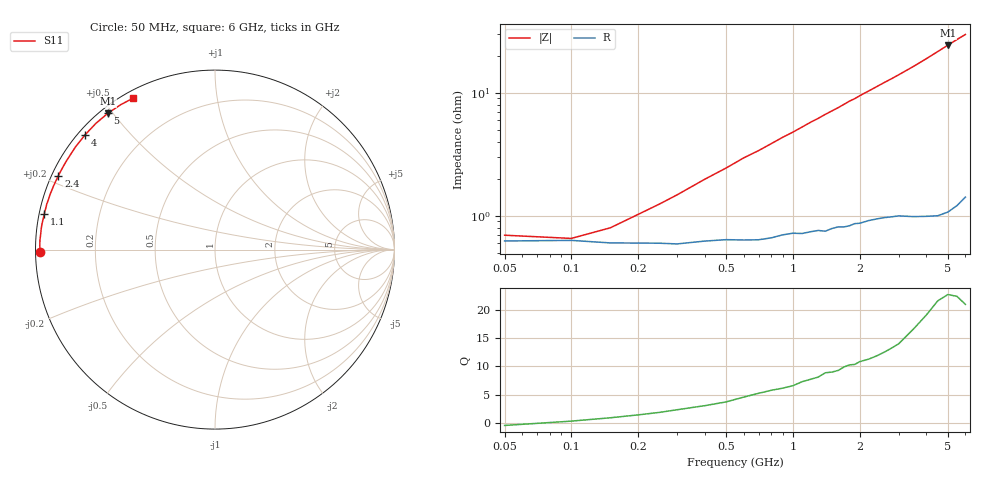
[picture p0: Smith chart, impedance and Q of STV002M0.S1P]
! SIEMENS Discrete & RF Semiconductors
! BA892
! Si PIN Diode in SCD-80
! IF = 2 mA
! S-Parameters:  September  1997
# GHz  S  MA  R  50
!  f  S11
! GHz  MAG  ANG
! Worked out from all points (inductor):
!   34 points, 50 MHz to 6 GHz, reference 50 ohm
!   read as one part to ground: L = 753 pH near 400 MHz
!   highest Q = 22.4 at 5 GHz (marker M1), where L = 774 pH
!   S11 on the Smith chart (normalised r, x): 50 MHz: 0.01, -0.01; 1.1 GHz: 0.01, +0.10; 2.4 GHz: 0.02, +0.22; 4 GHz: 0.02, +0.38; 5 GHz: 0.02, +0.49; 6 GHz: 0.03, +0.59
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0.05  0.9754 -179.3
0.1  0.9752 179.6
0.15  0.9763 178.8
0.2  0.9764 178.1
0.3  0.9768 176.9
0.6  0.9751 173.4
0.7  0.975 172.4
0.8  0.9741 171.3
0.9  0.9727 170.2
1  0.9719 169.2
1.1  0.9721 168.1
1.2  0.9712 167.0
1.3  0.9706 166.0
1.4  0.971 164.9
1.6  0.9688 162.9
1.8  0.9683 160.7
1.9  0.9672 159.8
2  0.9671 158.7
2.4  0.9648 154.7
2.6  0.9642 152.7
2.8  0.964 150.8
3  0.9637 148.8
3.5  0.9651 143.8
4  0.966 138.6
4.5  0.9669 133.3
5  0.966 128.1
5.5  0.9634 123.1
6  0.9591 118.5
